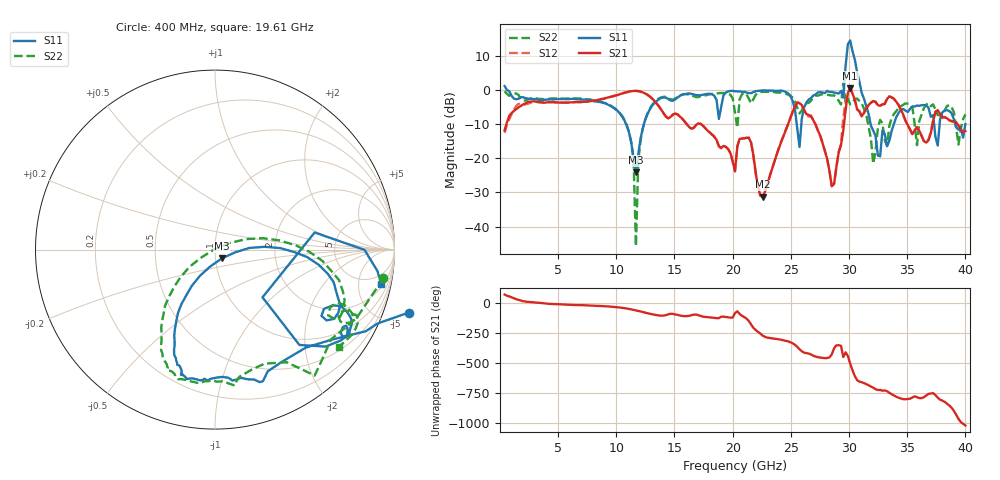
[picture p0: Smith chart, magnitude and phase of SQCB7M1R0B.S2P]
! Network Analyzer HP8722ES.07.66: Jul 25, 2000 Serial No. US39175408
! 26 Oct 2004  10:32:30
! Frequency  S11  S21  S12  S22
# HZ  S  DB R  50
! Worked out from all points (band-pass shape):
!   201 points, 400 MHz to 40 GHz, reference 50 ohm
!   highest |S21| = 0.45 dB at 30.1 GHz (marker M1); lowest = -31.3 dB at 22.58 GHz (marker M2)
!   |S21| within 3 dB of the highest: 8.989 GHz to 13.07 GHz (4.086 GHz wide, 37 % of centre); 29.84 GHz to 30.46 GHz (621.1 MHz wide, 2.06 % of centre)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
!   lowest |S11| = -24.2 dB at 11.69 GHz (marker M3), VSWR 1.13, Z = 53.7 - j5.28 ohm
!   |S11| at or under -10 dB: 10.83 GHz to 12.38 GHz (1.543 GHz wide, 13.3 % of centre); 31.85 GHz to 33.85 GHz (2.001 GHz wide, 6.09 % of centre); 39.13 GHz to end of sweep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
!   |S22| runs from -45.7 to 1.9 dB; largest |S21 - S12| = 0.16
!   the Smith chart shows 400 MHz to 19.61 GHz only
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4e8  1.11 -18.0  -11.81 73.3  -12.54 78.5  -0.43 -9.7
7.132e9  -2.87 -104.5  -3.53 -15.4  -3.58 -16.6  -2.74 -108.0
1.0894e10  -10.47 -122.1  -0.69 -43.0  -0.72 -43.6  -10.31 -137.8
1.1488e10  -20.08 -106.2  -0.33 -54.3  -0.31 -54.7  -20.86 -149.8
1.1686e10  -24.15 -52.2  -0.32 -58.7  -0.31 -59.1  -45.72 175.3
1.2082e10  -14.34 2.8  -0.53 -67.8  -0.49 -68.3  -14.83 18.8
1.3666e10  -2.73 -20.9  -4.84 -101.2  -4.86 -100.7  -2.50 -18.1
2.02e10  -0.41 -18.1  -23.88 -82.0  -23.73 -79.6  -6.64 -68.5
2.2576e10  -0.17 -20.4  -31.27 91.1  -31.13 89.8  -0.52 -14.2
2.5546e10  -11.07 -80.5  -3.82 -2.4  -3.64 -4.0  -5.26 -30.3
2.6932e10  -1.66 -15.1  -8.92 -76.7  -8.88 -77.3  -2.26 4.2
2.911e10  -1.08 -42.5  -18.34 11.2  -18.20 9.8  -3.18 -41.8
2.9506e10  -2.22 22.6  -11.93 -87.8  -8.29 -90.5  1.93 66.0
2.9704e10  7.04 -32.8  -5.89 -48.4  -3.64 -53.0  -3.76 -89.4
2.9902e10  13.35 -87.9  -0.89 -79.0  -0.90 -79.7  -2.59 -33.5
3.01e10  14.44 -125.3  0.45 -142.3  0.42 -144.2  -4.24 -51.1
3.0496e10  8.84 -164.6  -2.90 114.3  -2.81 112.7  -2.77 -70.2
3.0694e10  5.17 -14.9  -5.74 80.1  -5.66 79.4  -2.54 98.8
3.1288e10  -2.64 -46.7  -6.73 55.4  -6.74 55.0  -5.51 66.8
3.1486e10  -4.82 136.1  -5.38 46.4  -5.52 46.0  -7.29 -130.2
3.3466e10  -14.88 -145.6  -1.92 -24.8  -1.99 -25.0  -10.47 -82.8
4e10  -10.01 129.8  -12.04 62.4  -12.14 62.1  -7.19 122.2
